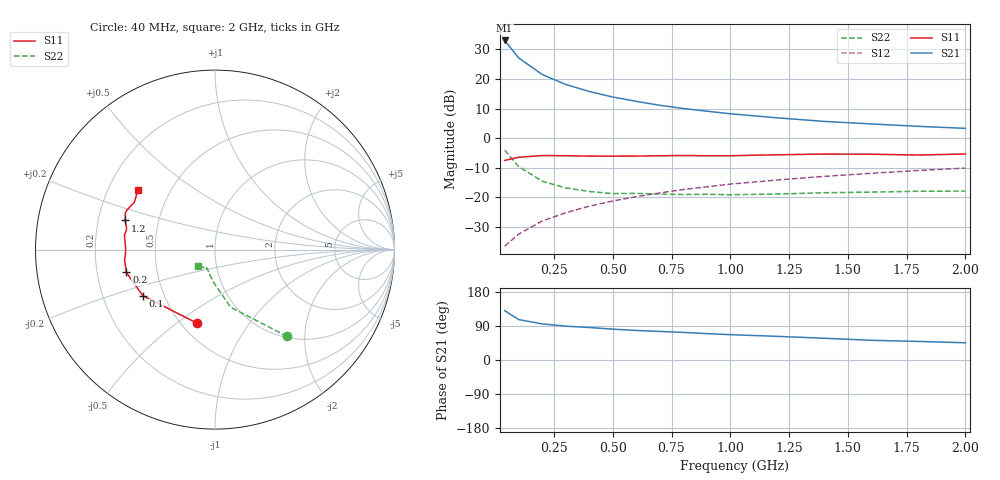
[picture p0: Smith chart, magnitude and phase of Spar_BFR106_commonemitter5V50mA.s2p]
! Filename:  BFR106C.S2P  Version:  2.0
! NXP part #: BFR106  Date: Jun 1990
! Bias condition: Vce=5V, Ic=50mA
#  MHz  S  MA  R  50
! Freq  S11  S21  S12  S22  !GUM [dB]
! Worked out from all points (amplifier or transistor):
!   16 points, 40 MHz to 2 GHz, reference 50 ohm
!   highest |S21| = 33.1 dB at 40 MHz (marker M1)
!   |S21| within 3 dB of that: start of sweep to 70.41 MHz
!   unconditionally stable (mu >= 1): 275 MHz to 1.999 GHz
!   at 200 MHz: K = 0.94, MSG = 24.8 dB, |S12| = -28.0 dB
!   at 800 MHz: K = 1.06, MAG = 12.2 dB, |S12| = -17.3 dB
!   at 2 GHz: K = 1.00, MSG = 6.7 dB, |S12| = -10.1 dB
!   S11 on the Smith chart (normalised r, x): 40 MHz: 0.60, -0.60; 100 MHz: 0.38, -0.25; 200 MHz: 0.33, -0.11; 1.2 GHz: 0.32, +0.14; 2 GHz: 0.33, +0.31
40  0.422 -103.7  44.96 130.4  0.015 61.2  0.629 -50.3
100  0.477 -147.4  22.74 106.7  0.024 60.8  0.332 -74.9
200  0.51 -165.6  11.96 95.3  0.04 69.2  0.188 -91.2
300  0.507 -173.6  8.115 89.3  0.055 70.5  0.145 -101.2
400  0.499 -177.5  6.179 85.8  0.071 72.5  0.126 -107.2
500  0.498 179.4  4.974 81.4  0.087 73.3  0.116 -111.2
600  0.5 177.1  4.207 78.0  0.103 73.2  0.117 -113.6
700  0.506 173.7  3.609 75.4  0.119 72.8  0.114 -114.3
800  0.511 170.6  3.188 72.8  0.136 72.3  0.112 -115.5
900  0.506 168.2  2.868 69.6  0.151 72.0  0.113 -114.6
1000  0.506 166.7  2.594 66.9  0.168 71.0  0.111 -116.5
1200  0.526 162.0  2.213 62.4  0.197 69.5  0.114 -120.9
1400  0.54 157.6  1.925 57.4  0.227 67.7  0.12 -124.1
1600  0.537 155.5  1.745 52.0  0.256 66.5  0.123 -126.7
1800  0.521 149.6  1.59 49.0  0.285 64.6  0.127 -129.8
2000  0.542 142.4  1.47 45.5  0.313 63.1  0.128 -136.2
